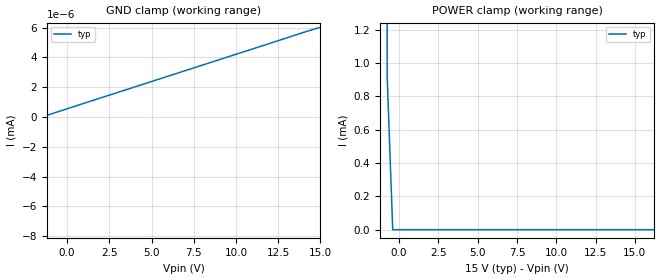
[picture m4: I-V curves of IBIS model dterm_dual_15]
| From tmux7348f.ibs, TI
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| dterm_dual_15
[Model]   dterm_dual_15
Model_type   Terminator
|   typ   min   max
C_comp   1.008417e-11   NA   NA
[Voltage Range]   15   NA   NA
[Temperature Range]   27   NA   NA
[Power Clamp Reference]   15   NA   NA
[GND Clamp Reference]   0   NA   NA
[GND Clamp]
|   Voltage   I(typ)   I(min)   I(max)
-20V      -1.414A    NA         NA
-15.05V   -11.62uA   NA         NA
-14.7V    -4.947nA   NA         NA
-14.34V   -4.692nA   NA         NA
15V       6.031nA    NA         NA
[POWER Clamp]
|   Voltage   I(typ)   I(min)   I(max)
-5V       1.414A     NA         NA
-1.111V   74.09mA    NA         NA
-757.6mV  919.6uA    NA         NA
-404mV    15.19nA    NA         NA
29.65V    -857.9pA   NA         NA
30V       -4.915uA   NA         NA
